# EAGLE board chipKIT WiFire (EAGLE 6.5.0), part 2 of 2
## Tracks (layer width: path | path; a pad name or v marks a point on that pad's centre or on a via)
AETXCLK/RPA14/SCL1/RA14  (via drill 0.23 pad 0.43)
  Top 0.127: v63.63,43.56 63.75,43.43 64.64,43.43 65.02,43.05 65.02,42.04 68.2,38.86 68.2,31.5 66.22,29.52 IC1.66 59.76,29.52 v59.69,29.59 | JP7.2 68.58,15.62 62.23,21.97 v62.23,22.35
  Bottom 0.127: v63.63,43.56 63.75,43.69 63.75,49.02 J7.1 | v59.69,29.59 59.69,29.46 60.2,28.96 60.2,24.38 60.83,23.75 60.83,23.37 61.85,22.35 v62.23,22.35
AETXEN/RPA15/SDA1/RA15  (via drill 0.23 pad 0.43)
  Top 0.127: IC3.33 26.16,32.26 v26.29,32.38 | v57.66,26.92 57.66,29.59 58.17,30.1 59.82,30.1 59.99,29.92 IC1.67
  Bottom 0.127: R21.1 26.42,32.51 v26.29,32.38 27.3,31.37 33.02,31.37 34.04,30.35 38.48,30.35 42.55,26.29 48.51,26.29 48.9,25.91 55.24,25.91 56.39,27.05 57.53,27.05 v57.66,26.92
AN2/C2INB/RPB2/RB2
  Top 0.203: IC1.23 46.42,24.32 45.21,23.11 45.21,19.68 51.82,13.08 54.61,13.08 55.5,12.19 66.04,12.19 71.37,6.86 71.88,6.86 J8.4
AN3/C2INA/RPB3/RB3
  Top 0.203: IC1.22 46.18,24.72 44.7,23.24 44.7,19.56 51.69,12.57 54.23,12.57 55.12,11.68 65.91,11.68 71.12,6.48 J8.2
AN4/C1INB/RB4
  Top 0.203: IC1.21 45.95,25.12 44.2,23.37 44.2,19.3 51.56,11.94 53.72,11.94 54.48,11.18 65.79,11.18 69.22,7.75 69.22,4.32 69.6,3.94 75.06,3.94 J8.6
AN6/ERXERR/AETXERR/RB11  (via drill 0.23 pad 0.43)
  Top 0.127: v82.04,44.32 81.28,43.56 76.96,43.56 v72.77,39.37 | IC1.35 52.9,22.93 53.59,23.62 53.59,27.18 52.9,27.87 52.9,29.28 53.85,30.23 v53.85,30.48
  Bottom 0.127: R25.1 82.05,44.33 v82.04,44.32 | v72.77,39.37 70.48,37.08 61.47,37.08 58.8,34.42 55.24,34.42 54.99,34.16 54.99,31.62 v53.85,30.48
AN8/ERXD1/AECOL/RB13  (via drill 0.23 pad 0.43)
  Top 0.203: v72.14,33.02 71.5,32.38 71.5,26.04 71.12,25.65 71.12,21.21 70.23,20.32 v67.69,20.32 | IC1.42 55.7,22.68 v55.75,22.73
  Bottom 0.203: v72.14,33.02 72.38,33.02 R11.1 | v55.75,22.73 56.26,23.24 60.45,23.24 61.85,21.84 62.99,21.84 64.52,20.32 v67.69,20.32
AN14/C1IND/ECOL/RPG6/SCK2/RG6  (via drill 0.23 pad 0.43)
  Top 0.127: v50.04,30.48 49.08,29.52 IC1.10
  Bottom 0.127: 77.98,44.97 R26.1 78.87,45.85 82.17,45.85 82.93,46.61 84.33,46.61 85.85,48.13 85.85,51.18 84.45,52.58 50.55,52.58 49.28,51.31 J7.11 50.42,49.66 50.42,47.75 49.28,46.61 46.74,46.61 44.83,44.7 44.83,40.51 44.96,40.39 44.96,34.8 48.39,31.37 49.15,31.37 v50.04,30.48 50.55,29.97 52.2,29.97 53.21,28.96 56.77,28.96 57.53,28.19 59.05,28.19 59.31,28.45 59.31,28.83 58.8,29.34 58.8,29.97 59.44,30.61 65.28,30.61 65.91,31.24 76.33,31.24 76.83,31.75 79.38,31.75 83.19,27.94 J9.3
AN23/AERXERR/RG15  (via drill 0.23 pad 0.43)
  Top 0.127: v85.09,45.85 85.34,45.59 85.34,39.12 84.58,38.35 73.03,38.35 71.5,39.88 71.5,41.53 68.83,44.2 58.04,44.2 57.28,43.43 56.39,43.43 v56.01,43.05 | IC1.1 48.29,33.12 v48.51,32.89
  Bottom 0.127: v85.09,45.85 R23.1 | v48.51,32.89 51.44,32.89 52.32,33.78 52.32,35.18 55.24,38.1 55.75,38.1 56.01,38.35 56.01,38.86 55.24,39.62 54.23,39.62 53.34,40.51 53.34,42.16 54.23,43.05 v56.01,43.05
AN25/AERXD0/RPE8/RE8  (via drill 0.23 pad 0.43)
  Top 0.127: v62.23,37.72 62.23,36.45 55.75,29.97 v55.75,28.32 | v50.8,27.56 50.55,27.56 49.31,26.32 IC1.18
  Bottom 0.127: J10.5 77.6,49.66 77.6,47.5 74.93,44.83 74.93,43.94 68.71,37.72 v62.23,37.72 | v55.75,28.32 55.75,28.19 54.61,27.05 51.69,27.05 51.44,27.3 51.05,27.3 v50.8,27.56
AN26/AERXD1/RPE9/RE9  (via drill 0.23 pad 0.43)
  Top 0.127: v64.39,42.93 64.39,42.42 62.74,40.77 62.74,36.45 56.39,30.1 56.39,28.19 v56.26,28.07 | v51.44,26.67 51.31,26.67 50.56,25.92 IC1.19
  Bottom 0.127: v64.39,42.93 64.39,49.15 J10.15 | v56.26,28.07 56.26,27.94 54.99,26.67 v51.44,26.67
AN32/AETXD0/RPD14/RD14  (via drill 0.23 pad 0.43)
  Top 0.127: v54.1,28.07 54.23,27.94 54.23,25.53 56.9,22.86 57.4,22.86 57.7,22.56 IC1.47
  Bottom 0.127: 49.4,48.26 J7.12 49.02,48.26 47.75,46.99 46.35,46.99 44.45,45.09 44.45,40.39 44.58,40.26 44.58,34.67 48.26,30.99 48.9,30.99 50.16,29.72 51.94,29.72 53.09,28.57 53.59,28.57 v54.1,28.07
AN33/AETXD1/RPD15/SCK6/RD15  (via drill 0.23 pad 0.43)
  Top 0.127: v53.47,28.07 53.98,28.57 54.36,28.57 54.61,28.32 54.61,25.78 57.28,23.11 57.53,23.11 58.1,22.54 IC1.48
  Bottom 0.127: J7.14 44.07,45.59 44.07,40.26 44.2,40.13 44.2,34.42 48.01,30.61 48.77,30.61 49.91,29.46 51.69,29.46 53.09,28.07 v53.47,28.07
AN45/C1INA/RPB5/RB5
  Top 0.203: IC1.20 45.59,25.52 43.69,23.62 43.69,19.05 51.44,11.3 52.83,11.3 53.59,10.54 53.59,9.4 54.61,8.38 64.14,8.38 69.98,2.54 J8.1
AVCC
  Top 0.254: IC1.30 50.9,20.8 C15.1
  pour Top (no thermals): 50.29,20.32 50.29,18.67 47.88,18.67 47.88,19.81 49.02,19.81 49.53,20.32
EBIA0/AN10/ERXD3/AETXD2/RPB15/OCFB/PMA0/RB15  (via drill 0.23 pad 0.43)
  Top 0.203: IC1.44 56.5,15.25 57.02,14.73 67.44,14.73 v75.18,6.99
  Bottom 0.203: J8.7 77.47,3.81 77.47,5.84 76.33,6.99 v75.18,6.99
EBIA1/AN9/ERXD2/AETXD3/RPB14/SCK3/PMA1/RB14  (via drill 0.23 pad 0.43)
  Top 0.127: J13.5 20.57,3.3 20.95,2.92 25.15,2.92 26.17,3.94 26.17,15.75 27.94,17.53 32,17.53 32.89,18.41 40.39,18.41 40.64,18.67 41.02,18.67 41.15,18.54 v41.27,18.54 | IC1.43 56.1,20.29 56.01,20.19 56.01,17.65 55.12,16.76 v52.7,16.76
  Bottom 0.127: v41.27,18.54 46.74,18.54 48.51,16.76 v52.7,16.76
EBIA2/AN11/C2INC/ERXCLK/EREFCLK/AERXCLK/AEREFCLK/RPG9/PMA2/RG9  (via drill 0.23 pad 0.43)
  Top 0.127: v50.67,30.48 50.67,29.34 50.29,28.96 50.29,28.07 49.15,26.92 v48.51,26.92 | 48.33,27.11 v48.51,26.92 | IC1.16 48.32,27.12 v48.51,26.92
  Bottom 0.127: J7.5 56.9,51.56 56.39,52.07 51.05,52.07 50.67,51.69 50.67,50.16 51.31,49.53 52.32,49.53 52.83,49.02 52.83,46.99 51.69,45.85 47.5,45.85 45.59,43.94 45.59,39.88 46.1,39.37 46.1,37.21 46.74,36.58 46.74,35.94 47.5,35.18 47.5,32.77 48.39,31.88 49.4,31.88 50.67,30.61 v50.67,30.48 | v48.51,26.92 49.15,26.29 51.05,26.29 51.18,26.16 51.94,26.16 52.07,26.29 55.12,26.29 56.26,27.43 58.8,27.43 59.69,28.32 59.69,28.96 59.18,29.46 59.18,29.84 59.44,30.1 77.09,30.1 77.34,29.84 78.23,29.84 JP5.1 JP5.2 80.9,27.18 82.68,25.4 J9.5
EBIA3/AN12/C2IND/ERXDV/ECRSDV/AERXDV/AECRSDV/RPG8/SCL4/PMA3/RG8  (via drill 0.23 pad 0.43)
  Top 0.127: IC1.12 48.24,28.72 48.39,28.57 48.9,28.57 v49.02,28.45
  Top 0.203: IC1.12 46.34,28.72 46.1,28.96 44.07,28.96 42.55,27.43 42.55,18.29 50.16,10.67 50.16,8.89 51.31,7.75 63.88,7.75 70.36,1.27 79.38,1.27 80.01,1.91 80.01,3.17 80.64,3.81 82.55,3.81 J8.11
  Bottom 0.127: J6.2 39.12,47.12 40.01,46.23 40.01,38.23 42.16,36.07 42.16,29.84 43.18,28.83 45.34,28.83 46.1,28.07 48.64,28.07 v49.02,28.45
EBIA4/AN13/C1INC/ECRS/RPG7/SDA4/PMA4/RG7  (via drill 0.23 pad 0.43)
  Top 0.127: v48.51,29.08 47.44,29.08 IC1.11
  Top 0.203: J8.9 81.28,2.29 79.76,0.76 70.1,0.76 63.75,7.11 51.05,7.11 49.4,8.76 49.4,10.41 41.78,18.03 41.78,27.69 43.43,29.34 46.23,29.34 46.44,29.12 IC1.11
  Bottom 0.127: J6.1 41.66,47.24 40.39,45.97 40.39,38.35 42.55,36.2 42.55,30.35 43.81,29.08 45.72,29.08 46.35,28.45 48.26,28.45 48.51,28.7 v48.51,29.08
EBIA5/AN34/PMA5/RA5  (via drill 0.23 pad 0.43)
  Top 0.127: IC1.2 43.77,32.72 40.51,29.46 40.51,24.77 v39.88,24.13
  Bottom 0.127: R27.1 25.03,25.53 31.62,25.53 32,25.91 33.78,25.91 34.04,25.65 38.35,25.65 v39.88,24.13
EBIA6/AN22/RPC1/PMA6/RC1  (via drill 0.23 pad 0.43)
  Top 0.127: IC1.6 48.52,31.12 48.77,31.37 53.98,31.37 54.74,32.13 57.28,32.13 57.91,32.77 58.17,32.77 60.45,35.05 60.45,35.69 61.59,36.83 61.59,42.93 61.72,43.05 v61.72,43.31
  Bottom 0.127: J7.4 59.44,48.64 60.33,49.53 62.23,49.53 63.12,48.64 63.12,45.21 61.72,43.81 v61.72,43.31
EBIA7/AN49/RPB9/PMA7/RB9  (via drill 0.23 pad 0.43)
  Top 0.203: IC1.33 52.1,16.61 53.59,15.11 55.75,15.11 56.64,14.22 67.06,14.22 v69.09,12.19
  Bottom 0.203: v69.09,12.19 74.93,6.35 74.93,3.81 J8.3
EBIA8/RPF5/SCL5/PMA8/RF5  (via drill 0.23 pad 0.43)
  Top 0.127: IC3.32 24.89,30.86 26.29,29.46 v27.81,29.46 | v57.91,25.91 57.91,26.04 58.42,26.54 58.42,28.19 58.29,28.32 58.29,28.83 58.59,29.12 IC1.65
  Bottom 0.127: v27.81,29.46 30.61,29.46 32.51,27.56 34.92,27.56 35.18,27.3 36.45,27.3 36.96,27.81 38.86,27.81 41.53,25.15 55.5,25.15 56.39,26.04 57.78,26.04 v57.91,25.91
EBIA9/RPF4/SDA5/PMA9/RF4  (via drill 0.23 pad 0.43)
  Top 0.127: IC3.7 22.35,51.56 v22.1,51.31 22.1,51.05 22.61,50.55 27.18,50.55 29.46,48.26 34.8,48.26 35.94,47.12 43.31,47.12 45.09,45.34 v48.01,45.34 | v58.8,28.7 60.78,28.7 IC1.64
  Bottom 0.127: v22.1,51.31 R14.1 | v48.01,45.34 48.01,39.12 50.67,36.45 50.67,33.66 50.29,33.27 49.02,33.27 48.77,33.53 48.13,33.53 47.88,33.27 47.88,32.89 48.51,32.26 50.42,32.26 53.34,29.34 57.66,29.34 58.29,28.7 v58.8,28.7
EBIA10/AN48/RPB8/PMA10/RB8
  Top 0.203: IC1.32 51.7,16.24 53.34,14.61 55.5,14.61 56.39,13.72 66.8,13.72 74.17,6.35 80.64,6.35 81.28,5.71 J8.10
EBIA11/AN7/ERXD0/AECRS/PMA11/RB12  (via drill 0.23 pad 0.43)
  Top 0.127: IC1.41 55.3,20.77 55.75,20.32 55.75,17.91 54.99,17.14 53.85,17.14 53.59,17.4 v53.09,17.4 | v43.69,15.24 40.13,15.24 39.5,15.88 35.81,15.88 32,12.06 v32,10.67
  Bottom 0.127: v53.09,17.4 53.09,17.27 53.21,17.14 53.21,16 52.45,15.24 v43.69,15.24 | v32,10.67 R35.1
  Bottom 0.203: R36.2 R35.1
EBIA12/AN21/RPC2/PMA12/RC2  (via drill 0.23 pad 0.43)
  Top 0.203: IC1.7 49.26,30.72 49.53,30.99 54.1,30.99 55.12,29.97 55.12,26.04 58.42,22.73 60.07,22.73 65.91,16.89 v65.91,15.37
  Bottom 0.203: v65.91,15.37 67.94,13.34 69.72,13.34 74.93,8.13 76.58,8.13 78.36,6.35 79.5,6.35 80.01,5.84 80.01,1.91 79.38,1.27 77.47,1.27 J8.5
EBIA13/CVREFOUT/AN5/RPB10/PMA13/RB10  (via drill 0.23 pad 0.43)
  Top 0.127: J13.7 18.29,4.89 18.29,3.43 19.3,2.41 25.65,2.41 28.37,5.13 28.37,15.29 30.1,17.02 40.01,17.02 v40.89,17.91 | IC1.34 52.5,18.87 v52.58,18.8
  Bottom 0.127: v40.89,17.91 40.77,18.03 40.77,18.8 41.02,19.05 46.99,19.05 48.01,18.03 51.82,18.03 v52.58,18.8
EBIA14/PMCS1/PMA14/RA4  (via drill 0.23 pad 0.43)
  Top 0.127: v57.66,24.64 58.17,25.15 58.17,25.53 58.42,25.78 58.42,26.04 58.67,26.29 58.67,27.18 59.02,27.52 IC1.61
  Bottom 0.127: v57.66,24.64 56.64,23.62 49.66,23.62 49.53,23.75 48.51,23.75 48.39,23.62 39.75,23.62 38.35,25.02 34.8,25.02 34.66,24.88 R29.1
EBIA15/RPD9/PMCS2/PMA15/RD9  (via drill 0.23 pad 0.43)
  Top 0.127: v13.46,32.38 IC3.23 13.5,31.71 14.22,30.99 19.18,30.99 23.11,27.05 v23.88,27.05 | v56.52,25.53 56.52,25.65 57.28,26.42 57.28,26.67 57.15,26.8 57.15,29.59 57.91,30.35 59.94,30.35 59.98,30.32 IC1.68
  Bottom 0.127: v13.46,32.38 13.46,33.01 R20.1 | v23.88,27.05 38.99,27.05 41.27,24.77 55.63,24.77 56.39,25.53 v56.52,25.53
EBICS0/SCL2/RA2  (via drill 0.23 pad 0.43)
  Top 0.127: v58.29,29.59 58.04,29.34 58.04,27.56 58.17,27.43 58.17,26.8 57.78,26.42 57.66,26.42 57.15,25.91 57.15,24.51 57.53,24.13 57.91,24.13 58.55,24.77 58.55,25.53 58.8,25.78 58.8,26.04 58.93,26.16 58.93,26.54 59.11,26.72 IC1.59
  Bottom 0.127: J7.8 56.52,46.1 56.52,42.8 55.37,41.66 55.37,40.01 56.39,38.99 56.39,38.35 55.88,37.85 55.5,37.85 54.74,37.08 54.74,36.45 52.96,34.67 52.96,33.66 52.07,32.77 52.07,31.11 53.47,29.72 58.17,29.72 v58.29,29.59
EBID0/PMD0/RE0
  Top 0.127: J10.2 81.79,46.23 78.11,46.23 76.45,44.58 56.52,44.58 55.5,43.56 55.5,42.55 55.75,42.29 55.75,40.51 53.09,37.85 53.09,36.32 52.9,36.14 IC1.91
EBID1/PMD1/RE1
  Top 0.127: J10.4 79.63,46.61 77.85,46.61 76.33,45.09 56.39,45.09 55.12,43.81 55.12,42.42 55.37,42.16 55.37,40.64 52.7,37.97 51.82,37.97 51.05,37.21 51.05,36.45 51.31,36.2 51.56,36.2 51.7,36.05 IC1.94
EBID2/PMD2/RE2
  Top 0.127: 76.07,45.59 77.22,46.74 77.47,46.74 78.74,48.01 J10.6 | 50.67,45.59 48.9,43.81 46.35,43.81 45.47,42.93 45.47,40.01 47.62,37.85 48.39,37.85 49.78,36.45 49.78,36.2 50.1,35.88 IC1.98
  Top 0.203: 50.67,45.59 76.07,45.59
EBID3/RPE3/PMD3/RE3
  Top 0.127: J10.8 76.2,47.5 74.8,46.1 50.42,46.1 48.51,44.2 46.1,44.2 44.83,42.93 44.83,40.13 47.62,37.34 48.26,37.34 49.7,35.9 IC1.99
EBID4/AN18/PMD4/RE4
  Top 0.127: J10.10 73.66,47.24 73.03,46.61 50.29,46.61 48.39,44.7 45.85,44.7 44.45,43.31 44.45,40.01 47.62,36.83 48.26,36.83 49.3,35.79 IC1.100
EBID5/AN17/RPE5/PMD5/RE5  (via drill 0.23 pad 0.43)
  Top 0.127: v52.96,32.51 52.77,32.32 IC1.3
  Bottom 0.127: J10.12 70.74,47.88 70.74,43.81 67.44,40.51 63.5,40.51 57.78,34.8 55.12,34.8 54.23,33.91 54.23,32.38 53.85,32 53.47,32 v52.96,32.51
EBID6/AN16/PMD6/RE6  (via drill 0.23 pad 0.43)
  Top 0.127: IC1.4 48.43,31.92 48.51,32 53.21,32 v53.72,32.51
  Bottom 0.127: J10.14 67.82,47.5 67.82,43.31 66.17,41.66 63.12,41.66 60.2,38.73 57.78,38.73 56.9,37.85 56.9,36.32 55.75,35.18 54.86,35.18 53.72,34.04 v53.72,32.51
EBID7/AN15/PMD7/RE7  (via drill 0.23 pad 0.43)
  Top 0.127: v60.07,39.88 59.69,39.5 59.69,34.67 58.04,33.02 57.15,33.02 56.64,32.51 54.61,32.51 53.85,31.75 48.64,31.75 48.41,31.52 IC1.5
  Bottom 0.127: v60.07,39.88 62.61,42.42 64.64,42.42 65.15,42.93 65.15,47.37 J10.16
EBID8/RPG0/PMD8/RG0
  Top 0.127: IC1.88 54.1,34.16 53.98,34.04 53.98,33.91 53.85,33.78 52.2,33.78 51.82,33.4 49.78,33.4 48.9,34.29 48.9,34.54 42.04,41.4 36.83,41.4 35.05,43.18 31.5,43.18 28.57,40.26 28.57,31.84 IC3.35
EBID9/ETXERR/RPG1/PMD9/RG1  (via drill 0.23 pad 0.43)
  Top 0.127: IC3.20 v9.65,32.38 11.43,34.16 27.69,34.16 28.07,33.78 28.07,31.11 28.32,30.86 30.35,30.86 30.86,31.37 30.86,39.24 32.51,40.89 38.35,40.89 41.78,37.47 43.94,37.47 44.07,37.59 44.83,37.59 47.5,34.92 47.88,34.92 49.66,33.15 51.94,33.15 52.32,33.53 54.1,33.53 54.5,33.93 IC1.87
  Bottom 0.127: R19.1 v9.65,32.38
EBID10/ETXD0/RPF1/PMD10/RF1  (via drill 0.23 pad 0.43)
  Top 0.127: IC1.86 54.9,35.78 54.61,36.07 54.36,36.07 53.98,36.45 53.98,37.72 56.01,39.75 57.28,39.75 58.04,40.51 58.04,41.78 v57.66,42.16
  Bottom 0.127: J7.6 56.9,47.62 57.66,46.86 57.66,43.18 57.4,42.93 57.4,42.42 v57.66,42.16
EBID11/ETXD1/RPF0/PMD11/RF0  (via drill 0.23 pad 0.43)
  Top 0.127: v55.5,38.61 54.48,37.59 54.48,36.7 55.3,35.88 IC1.85 55.3,34.11 v55.5,33.91
  Bottom 0.127: J7.9 51.94,50.8 53.21,49.53 53.21,43.81 52.96,43.56 52.96,40.26 53.98,39.24 54.86,39.24 v55.5,38.61 | J9.1 81.41,30.48 79.63,32.26 76.07,32.26 75.44,31.62 64.52,31.62 63.88,30.99 61.34,30.99 60.33,32 56.52,32 55.5,33.02 v55.5,33.91
EBID12/ETXD2/RPD12/PMD12/RD12  (via drill 0.23 pad 0.43)
  Top 0.127: v46.99,33.78 48.26,33.78 49.4,32.64 52.2,32.64 52.58,33.02 56.64,33.02 57.02,33.4 57.4,33.4 57.7,33.7 IC1.79
  Bottom 0.127: J7.10 49.78,46.23 46.99,46.23 45.21,44.45 45.21,40.64 45.34,40.51 45.34,37.47 45.72,37.08 45.72,34.67 46.61,33.78 v46.99,33.78
EBID13/ETXD3/PMD13/RD13  (via drill 0.23 pad 0.43)
  Top 0.127: IC1.80 57.3,34.06 56.77,33.53 55.75,33.53 55.63,33.4 54.36,33.4 54.23,33.27 52.45,33.27 52.07,32.89 49.53,32.89 48.13,34.29 43.69,34.29 39.37,29.97 39.37,21.34 v40.26,20.45
  Bottom 0.127: R37.1 50.29,7.37 50.29,9.65 48.64,11.3 46.86,11.3 40.26,17.91 v40.26,20.45
EBID14/ETXEN/RPD2/PMD14/RD2  (via drill 0.23 pad 0.43)
  Top 0.127: v58.93,39.24 58.67,38.99 58.67,36.07 58.5,35.9 IC1.77
  Bottom 0.127: v58.93,39.24 59.05,39.12 60.07,39.12 62.99,42.04 65.41,42.04 66.55,43.18 66.55,46.74 67.31,47.5 67.31,49.53 J10.13
EBID15/ETXCLK/RPD3/PMD15/RD3  (via drill 0.23 pad 0.43)
  Top 0.127: IC1.78 58.1,35.88 58.29,36.07 58.29,40.13 58.42,40.26 58.42,42.29 v58.17,42.55
  Bottom 0.127: J7.3 59.31,50.8 58.17,49.66 v58.17,42.55
EBIOE/AN19/RPC4/PMRD/RC4
  Top 0.127: J13.3 22.77,4.03 23.24,3.56 25.27,3.56 25.78,4.06 25.78,16.26 27.69,18.16 31.75,18.16 32.51,18.92 40.13,18.92 41.27,20.07 41.27,28.45 42.75,29.92 IC1.9
EBIRDY1/SDA2/RA3  (via drill 0.23 pad 0.43)
  Top 0.127: IC1.60 61.78,27.12 61.98,26.92 66.29,26.92 69.22,29.84 69.22,34.29 68.96,34.54 v68.96,40.51
  Bottom 0.127: J10.9 72.39,49.53 72.39,44.7 68.96,41.27 v68.96,40.51
EBIRDY2/RPF8/SCL3/RF8  (via drill 0.23 pad 0.43)
  Top 0.127: v59.69,26.29 60.77,26.29 IC1.58 61.63,26.32 61.85,26.54 66.55,26.54 69.85,29.84 69.85,33.53 70.99,34.67 75.56,34.67 76.2,35.31 76.2,37.47 v75.82,37.85
  Bottom 0.127: R8.2 20.45,18.29 21.46,19.3 21.46,21.46 21.72,21.72 21.72,25.15 22.73,26.16 38.48,26.16 40.64,24 56.26,24 57.4,25.15 59.31,25.15 59.82,25.65 59.82,26.16 v59.69,26.29 | J10.3 80.01,49.53 80.01,47.62 79.25,46.86 77.72,46.86 75.69,44.83 75.69,37.97 v75.82,37.85
EBIRDY3/RPF2/SDA3/RF2  (via drill 0.23 pad 0.43)
  Top 0.127: v59.31,25.78 59.82,25.78 59.94,25.91 60.79,25.91 IC1.57 61.73,25.92 61.98,26.16 66.8,26.16 70.36,29.72 70.36,32.38 71.75,33.78 75.69,33.78 76.71,34.8 v76.71,37.85
  Bottom 0.127: J10.1 82.55,49.53 82.55,47.62 81.28,46.35 77.98,46.35 76.2,44.58 76.2,41.02 76.71,40.51 v76.71,37.85 | R7.2 18.04,20.58 19.18,21.72 20.7,21.72 21.08,22.1 21.08,25.27 22.35,26.54 38.86,26.54 41.02,24.38 56.13,24.38 57.15,25.4 58.93,25.4 v59.31,25.78
EBIWE/AN20/RPC3/PMWR/RC3
  Top 0.127: J13.2 24.13,5.63 24.13,5.97 25.02,6.86 25.02,16.26 24.51,16.76 22.61,16.76 22.48,16.89 R22.1 22.6,17.53 25.91,17.53 27.3,18.92 31.75,18.92 32.26,19.43 40.01,19.43 40.89,20.32 40.89,28.7 42.51,30.32 IC1.8
EMDC/AEMDC/RPD11/RD11  (via drill 0.23 pad 0.43)
  Top 0.127: v66.55,30.73 66.17,30.35 63.63,30.35 63.25,30.73 62.74,30.73 62.35,31.12 IC1.70 v59.69,31.11
  Bottom 0.127: v66.55,30.73 76.71,30.73 77.09,31.11 79.12,31.11 81.66,28.57 81.66,27.94 82.8,26.8 85.22,26.8 J9.4 | J7.7 54.48,50.8 55.63,49.66 55.63,47.88 56.9,46.61 56.9,42.67 55.88,41.66 55.88,40.01 56.77,39.12 56.77,38.35 56.01,37.59 55.63,37.59 55.12,37.08 55.12,36.07 53.34,34.29 53.34,33.53 52.45,32.64 52.45,31.62 53.34,30.73 53.34,30.35 53.72,29.97 54.23,29.97 55.37,31.11 v59.69,31.11
EMDIO/AEMDIO/RPD0/RTCC/INT0/RD0  (via drill 0.23 pad 0.43)
  Top 0.127: v67.56,38.35 67.06,37.85 67.06,33.15 65.02,31.11 62.87,31.11 62.46,31.52 IC1.71
  Bottom 0.127: J10.7 75.06,49.66 75.06,47.24 73.91,46.1 73.91,44.7 v67.56,38.35
FT3V3  (via drill 0.23 pad 0.43)
  Top 0.508: 12.32,25.02 12.32,22.61 12.95,21.97 14.86,21.97 v16.26,20.57 | 12.32,25.02 12.57,25.27 12.57,26.8 11.94,27.43 11.94,29.59 12.83,30.48 v15.75,30.48 v16.76,30.48 | 12.32,25.02 11.05,25.02 v10.16,25.91
  Bottom 0.127: R9.2 v16.76,30.48 | R10.2 v15.75,30.48
  Bottom 0.254: IC2.16 10.96,25.63 C13.1 v10.17,25.92 v10.16,25.91 | IC2.1 15.72,20.59 C11.1 16.25,20.57 v16.26,20.57
GND  (via drill 0.23 pad 0.43)
  Top 0.127: C20.2 v63,31.76 v62.99,31.75 | C19.2 v63,34.79 v62.99,34.8
  Top 0.203: IC7.2 61.66,16.58 61.72,16.51
  Top 0.254: IC3.30 22.35,31.5 22.1,31.24 C21.2 21.84,30.23 v21.84,29.97 | IC3.18 8.38,51.94 8.64,51.69 v8.64,51.56 | IC3.10 v18.54,51.44 | IC3.1 v29.97,51.44 | IC3.19 v8.38,32.38 | IC3.25 v16,32.38 | IC3.28 v19.81,32.38 | IC3.36 v29.97,32.38 | C15.2 | C15.2 v51.05,19.44 v51.05,19.43 | C14.2 51.05,18.79 v50.8,18.54 | C15.2 51.05,20.31 51.3,20.57 IC1.31 | C6.2 | C6.2 v53.09,19.44 v53.09,19.43 | C8.2 | v19.94,3.68 19.47,4.15 J13.6 | v52.32,37.08 52.32,36.95 C3.2 52.5,36.63 IC1.92 | IC1.84 55.7,36.51 C2.2 55.75,36.95 v55.75,37.08 | IC1.53 62.41,24.32 C1.2 62.73,24 v62.99,24 | IC1.63 62.24,28.32 C10.2 62.73,28.32 v62.99,28.32 | IC1.13 45.84,28.32 C4.2 45.6,28.32 v45.21,28.32 | IC1.36 53.3,20.15 C6.2 | IC1.45 56.9,20.07 C8.2 | 61.59,33.15 v61.72,33.27 61.57,33.12 IC1.75 | C8.2 v57.02,19.43
  Top 0.305: v62.23,16.51 61.72,16.51 | C17.2 v57.78,16.38
  Top 1.27: 5.08,20.19 J1.S3 J1.S2 5.08,29.09 | 5.08,20.19 J1.S4 | J1.S1 5.08,29.09 | J1.S5 5.08,29.09 | J1.S6 5.08,20.19
  Route2 1.524: 4.32,12.19 J15.2 4.32,4.45 5.84,2.92 J15.3
  Bottom 0.127: C5.2 R2.1 v10.67,29.46 | R30.1 v23.37,25.4 | R32.1 v32.77,25.4 | R15.1 v13.2,51.3 v13.21,51.31 | R17.1 v79.49,15.76 v79.5,15.75
  Bottom 0.203: Q2.1 v79.12,42.55 | Q2.4 80.45,44.13 v80.52,44.2
  Bottom 0.254: IC2.24 15.72,26.52 v15.88,26.67 | IC2.26 16.74,25.13 v16.76,25.15 | C13.2 v10.17,26.92 v10.16,26.92 | IC2.4 v14.22,21.09 v14.22,21.08 | C11.2 16,19.81 v16.13,19.81 | IC2.17 11.97,26.13 v11.81,26.29 | R41.1 v35.31,22.1 | IC2.20 13.72,26.94 C9.2 13.96,27.68 v13.97,27.69 | C7.2 14.35,28.7 | 14.35,28.7 v13.97,28.32 | C23.2 v8.64,51.55 v8.64,51.56 | D2.2 v31.5,41.02 | R36.1 31.11,8.89 v31.88,8.13 | 14.35,28.7 14.35,28.83 14.1,29.08 v13.97,29.08 | Q1.1 v83.19,42.55 | Q1.4 84.52,44.13 v84.58,44.2 | v19.68,48.77 19.68,49.13 C25.2 18.92,49.16 v18.92,48.77 | v4.7,33.53 4.7,33.92 C26.2 5.08,34.29 5.46,33.91 v5.46,33.53 | C27.2 20.07,3.55 v19.94,3.68 | D1.1 50.78,28.21 v50.8,28.19 | C12.2 61.46,33.27 v61.72,33.27
  Bottom 1.27: J11.S3 J11.S1 J11.S2 J11.S4 87.25,13.27 v87.25,11.18
  other vias: 6.48,22.48 6.99,21.97 85.22,15.24 84.2,15.24 13.21,24.64 14.73,24.64 13.21,23.11 14.73,23.11 7.49,22.48 8,21.97 8.51,22.48 13.34,10.92 13.34,11.94 13.34,12.95 13.34,13.72 13.34,14.61 14.22,10.92 14.22,11.94 14.22,12.95 22.73,7.24 22.73,6.48 23.75,6.48 32.26,20.45 32.77,20.07 33.4,20.45 33.15,17.78 34.04,17.78 36.83,17.91 36.07,17.91 37.85,14.99 37.85,13.97 35.31,17.91 37.34,14.48 37.34,13.34 37.85,12.95 37.34,12.32 67.94,25.65 67.94,26.29 83.57,15.75 83.57,14.61 84.84,14.61 81.03,14.22 81.03,13.34 80.52,18.54 81.92,18.54 86.87,11.81 87.63,11.81
  pour Top (no thermals): 6.22,23.37 9.02,23.37 9.02,21.72 6.22,21.72
  pour Bottom (no thermals): 85.47,16 83.06,16 83.06,14.22 85.47,14.22
  pour Top (no thermals): 5.21,5.59 5.21,9.65 4.7,10.16 3.94,10.16 3.43,9.65 3.43,5.59 3.94,5.08 4.7,5.08
  pour Top (no thermals): 5.33,2.03 9.4,2.03 9.91,2.54 9.91,3.3 9.4,3.81 5.33,3.81 4.83,3.3 4.83,2.54
  pour Bottom (no thermals): 3.43,9.65 3.94,10.16 4.7,10.16 5.21,9.65 5.21,5.59 4.7,5.08 3.94,5.08 3.43,5.59
  pour Bottom (no thermals): 4.83,3.3 5.33,3.81 9.4,3.81 9.91,3.3 9.91,2.54 9.4,2.03 5.33,2.03 4.83,2.54
  pour Bottom (isolate 0.305, rank 2, no thermals): 13.08,9.27 15.11,9.27 15.11,14.99 13.08,14.99
  pour Bottom (no thermals): 22.48,7.49 22.61,7.62 24,7.62 24,5.59 22.48,5.59
  pour Bottom (isolate 0.305, rank 2, no thermals): 32,22.48 32,19.81 32.77,19.81 32.89,19.68 32.89,17.14 37.21,17.14 37.34,17.02 37.34,14.73 37.21,14.61 35.05,14.61 35.05,12.19 38.61,12.19 38.61,18.29 37.08,19.81 35.18,19.81 35.18,18.41 34.92,18.16 33.78,18.16 33.66,18.29 33.66,22.48
  pour Route2 (isolate 0.305): 12.57,0 12.57,11.18 0,11.18 0,35.94 11.81,35.94 11.81,50.93 8.26,50.93 8.26,53.34 88.9,53.34 88.9,0
  pour Route2 (no thermals): 3.43,9.65 3.94,10.16 4.7,10.16 5.21,9.65 5.21,5.59 4.7,5.08 3.94,5.08 3.43,5.59
  pour Route2 (no thermals): 4.83,2.54 4.83,3.3 5.33,3.81 9.4,3.81 9.91,3.3 9.91,2.54 9.4,2.03 5.33,2.03
  pour Bottom (rank 2, no thermals): 68.2,25.4 68.2,26.42 66.93,26.42 66.93,25.4
  pour Bottom (no thermals): 80.64,14.73 80.64,12.7 82.55,12.7 82.55,14.73
  pour Bottom (rank 2, no thermals): 80.14,18.92 80.14,18.16 82.17,18.16 82.17,18.92
  pour Route15 (no thermals): 5.21,5.59 5.21,9.65 4.7,10.16 3.94,10.16 3.43,9.65 3.43,5.59 3.94,5.08 4.7,5.08
  pour Route15 (no thermals): 5.33,2.03 9.4,2.03 9.91,2.54 9.91,3.3 9.4,3.81 5.33,3.81 4.83,3.3 4.83,2.54
N$1
  Bottom 0.406: C24.1 JP6.1
N$14
  Bottom 0.127: C16.2 17.78,23.87 17.78,29.46 22.23,33.91 24.89,33.91 26.16,35.18 29.97,35.18 30.35,35.56 35.69,35.56 36.96,34.29 39.37,34.29 JP2.2
N$17
  Top 0.203: IC1.49 58.5,20.62 59.05,20.07 60.83,20.07 61.38,19.52 IC7.3
N$18
  Top 0.127: X2.2 65.79,33.91 65.41,34.29 64.9,34.29 64.64,34.04 64.64,33.4 64.26,33.02 63.76,33.02 C20.1 62.99,32.26 62.87,32.26 62.48,31.88 61.47,31.88 61.42,31.92 IC1.72
N$19
  Top 0.127: IC1.73 61.53,32.32 61.72,32.13 62.36,32.13 62.48,32.26 R13.2
N$20
  Top 0.127: X2.1 65.79,35.05 65.41,34.67 64.77,34.67 64.26,34.16 64.26,33.53 64.14,33.4 63.88,33.4 C19.1 62.5,33.79 R13.1
N$21  (via drill 0.23 pad 0.43)
  Top 0.127: IC1.15 46.44,27.52 v46.35,27.43
  Bottom 0.127: D1.3 46.48,27.56 v46.35,27.43 46.1,27.18 44.96,27.18 44.32,27.81 R4.1
N$22
  Bottom 0.127: R24.2 79.63,44.58 79.63,43.43 79.88,43.18 Q2.5
N$23
  Bottom 0.127: Q2.3 77.85,43.81 77.6,43.56 77.6,40.64 78.49,39.75 79.5,39.75 79.76,40.01 79.76,40.64 R33.1
N$25
  Bottom 0.127: R16.1 82.04,16.26 82.04,16.89 81.34,17.59 IC4.3 80.33,17.59 79.63,18.29 77.6,18.29 76.58,19.3 69.98,19.3 JP7.1
N$26  (via drill 0.23 pad 0.43)
  Top 0.127: v80.9,40.77 80.9,41.01 LD2.C
  Bottom 0.127: R33.2 v80.9,40.77
N$27
  Bottom 0.127: BTN3.1B 38.14,39.54 38.23,39.62 R6.1 37.47,40.64 37.08,41.02 37.08,44.11 BTN3.2B
N$28  (via drill 0.23 pad 0.43)
  Top 0.127: LD1.C 78.75,41.39 79.12,41.02 v79.12,40.77
  Bottom 0.127: v79.12,40.77 v79.11,40.77 R34.2
N$29  (via drill 0.23 pad 0.43)
  Top 0.127: IC3.26 17.27,31.75 16.89,32.13 v16.89,32.51
  Bottom 0.127: v16.89,32.51 16.89,32.65 R18.1
N$30
  Bottom 0.127: J17.5 49.28,7.37 R37.2
N$31
  Bottom 0.127: Q2.2 79.12,43.18 79.25,43.31 79.25,44.7 R26.2
N$32
  Bottom 0.127: 80.26,42.55 Q2.6 80.39,42.55 79.24,41.39 R34.1
N$33  (via drill 0.23 pad 0.43)
  Top 0.254: J1.2 9.11,25.44 v9.14,25.4
  Bottom 0.254: IC2.15 9.93,25.13 9.65,25.4 v9.14,25.4
N$34
  pour Bottom (rank 2, no thermals): 23.62,17.65 23.62,14.61 28.7,14.61 30.99,12.32 33.02,12.32 33.02,14.61 32.64,14.61 32.64,16.64 31.5,16.64 31.24,16.38 30.23,16.38 29.97,16.64 29.97,17.4 29.72,17.65
N$35
  Bottom 0.305: 30.75,16.89 C30.1 D5.C | 32.32,18.73 31.88,18.29 30.75,18.29
  Bottom 0.508: IC5.1 32.32,18.73 | 30.75,18.29 D5.C
N$36
  pour Bottom (isolate 0.305, rank 2, no thermals): 20.57,6.86 22.1,6.86 22.1,7.62 22.48,8 24,8 24,10.29 22.86,10.29 22.86,9.53 22.61,9.27 20.57,9.27
N$37  (via drill 0.23 pad 0.43)
  Top 0.254: J1.3 9.14,24.64 v9.27,24.77
  Bottom 0.254: IC2.14 9.41,24.63 v9.27,24.77
N$38
  Bottom 0.254: IC5.3 34.22,19.62 34.29,19.68 R40.1 R41.2
N$39
  pour Bottom (isolate 0.305, rank 3, no thermals): 17.78,3.56 17.78,8.64 17.4,9.02 13.08,9.02 13.08,3.56
N$40
  Bottom 0.203: R11.2 VR1.2
N$41
  Bottom 0.127: IC2.30 18.02,23.13 18.29,22.86 18.29,22.34 R7.1
N$43
  Bottom 0.127: IC2.2 15.22,21.06 15.11,20.95 15.11,19.18 15.49,18.8 R8.1
N$45  (via drill 0.23 pad 0.43)
  Top 0.127: IC3.16 10.92,52.07 v11.81,51.18
  Bottom 0.127: v11.81,51.18 v11.82,51.18 R15.2
N$47
  Bottom 0.127: IC2.18 12.72,26.4 12.19,26.92 12.19,27.44 C5.1 R2.2 9.67,28.95 R1.1
N$51  (via drill 0.23 pad 0.43)
  Top 0.127: LD3.C 82.68,41.02 v82.68,40.77
  Bottom 0.127: v82.68,40.77 82.67,40.77 R31.2
N$52
  Bottom 0.127: IC2.8 12.22,20.73 10.54,19.05 7.87,19.05 J4.1
N$53
  Bottom 0.127: IC2.31 17.51,22.63 C16.1
N$54
  Bottom 0.127: IC2.6 13.22,18.43 12.7,17.91 12.7,16.76 12.06,16.13 9.78,16.13 J4.2
N$55
  Bottom 0.127: IC2.7 12.72,18.56 11.43,17.27 J4.3
N$56
  Bottom 0.127: IC2.3 14.72,17.77 14.22,17.27 J4.4
N$57  (via drill 0.23 pad 0.43)
  Top 0.127: v15.75,27.56 15.86,27.56 LD5.C
  Bottom 0.127: IC2.22 14.72,26.53 v15.75,27.56
N$58  (via drill 0.23 pad 0.43)
  Top 0.127: v14.99,27.56 LD6.C
  Bottom 0.127: IC2.21 14.22,26.54 14.99,27.3 v14.99,27.56
N$59  (via drill 0.23 pad 0.43)
  Top 0.127: v17.14,29.34 16.88,29.34 LD5.A
  Bottom 0.127: R9.1 16.77,28.96 v17.14,29.34
N$60  (via drill 0.23 pad 0.43)
  Top 0.127: v15.37,29.21 15.37,29.32 LD6.A
  Bottom 0.127: R10.1 15.61,28.96 v15.37,29.21
N$62
  Bottom 0.127: IC4.4 78.49,17.28 R17.2 77.85,16.26 77.6,16 77.6,15.49 76.96,14.86 74.68,14.86 JP8.1
N$63  (via drill 0.23 pad 0.43)
  Top 0.127: LD4.C 84.09,41.39 84.45,41.02 v84.45,40.77
  Bottom 0.127: v84.45,40.77 R28.2
N$64
  Bottom 0.127: Q1.6 84.33,42.55 83.82,42.04 82.94,42.04 R31.1
N$65
  Bottom 0.127: Q1.3 82.17,43.81 81.92,43.56 81.92,42.42 81.53,42.04 81.53,40.13 81.92,39.75 82.93,39.75 83.19,40.01 83.19,40.51 R28.1
N$66
  Bottom 1.016: J12.1 78.47,13.52 C22.1
  pour Route15 (isolate 0.305, no thermals): 71.75,23.11 71.12,22.48 71.12,20.95 73.03,19.05 73.03,14.73 75.18,12.57 76.96,12.57 76.96,14.48 75.95,14.48 75.31,15.11 75.31,19.68 73.79,21.21 73.79,22.48 73.15,23.11
N$67
  Bottom 0.127: Q1.2 83.06,43.18 83.31,43.43 83.31,44.7 R25.2
N$69
  Bottom 0.127: R23.2 83.69,44.58 83.69,43.43 83.95,43.18 Q1.5
N$71
  Bottom 0.127: 32.74,23.91 R32.2 | R32.2 R29.2 33.81,23.91 BTN2.2A | BTN2.1A 29.29,23.88 R32.2
N$72  (via drill 0.23 pad 0.43)
  Top 0.127: v22.73,23.88 19.9,23.88 BTN1.1A
  Bottom 0.127: v22.73,23.88 22.77,23.91 23.34,23.91 R30.2 R27.2 24.41,23.91 BTN1.2A
P32_PGC  (via drill 0.23 pad 0.43)
  Top 0.127: v37.85,24 37.85,30.48 35.56,32.77 35.56,35.1 JP1.5 | IC1.26 49.3,20.73 v49.28,20.7
  Bottom 0.127: D2.5 30.85,39.64 33.27,37.21 33.45,37.21 JP1.5 | v37.85,24 37.85,23.75 39.24,22.35 48.26,22.35 48.64,21.97 48.95,21.97 IC1.26 49.3,20.73 v49.28,20.7
P32_PGD  (via drill 0.23 pad 0.43)
  Top 0.127: JP1.4 34.42,39.37 36.2,37.59 36.2,33.02 38.35,30.86 v38.35,24.38 | v48.77,22.61 48.9,22.73 49.53,22.73 49.7,22.56 IC1.27
  Bottom 0.127: D2.4 33.87,39.74 JP1.4 | v38.35,24.38 38.35,23.88 39.24,22.99 48.39,22.99 v48.77,22.61
P32_RST  (via drill 0.23 pad 0.43)
  Top 0.127: JP2.1 38.1,33.78 38.99,32.89 v38.99,20.32
  Bottom 0.127: JP1.1 32.38,45.54 32.38,41.91 32.15,41.67 D2.3 32.15,41.51 33.02,40.64 35.94,40.64 36.45,40.13 36.45,36.2 37.08,35.56 JP2.1 | v38.99,20.32 38.99,18.54 46.61,10.92 46.61,9.27 46.86,9.02 46.86,6.6 48.9,4.57 50.8,4.57 52.83,2.54 J5.3 | R4.2 42.8,27.81 41.78,28.83 41.78,35.94 40.89,36.83 40.26,36.83 38.99,35.56 JP2.1 | JP2.1 38.1,36.7 39.23,37.84 R6.2 R5.1
PGEC1/AN1/RPB1/RB1  (via drill 0.23 pad 0.43)
  Top 0.203: IC1.24 46.53,23.92 45.59,22.99 45.59,19.94 51.94,13.59 54.86,13.59 55.75,12.7 v66.29,12.7
  Bottom 0.203: v66.29,12.7 69.47,12.7 74.55,7.62 76.33,7.62 78.74,5.21 J8.8
PGED1/AN0/RPB0/RB0  (via drill 0.23 pad 0.43)
  Top 0.203: IC1.25 46.76,23.52 46.1,22.86 46.1,20.19 52.2,14.1 55.12,14.1 56.01,13.21 66.55,13.21 67.06,12.7 v67.06,12.06
  Bottom 0.203: v67.06,12.06 67.06,3.81 70.1,0.76 81.41,0.76 82.55,1.91 82.55,3.81 J8.12 82.04,6.86 78.49,6.86 76.58,8.76 75.06,8.76 71.37,12.45 JP8.2
RPD1/SCK1/RD1  (via drill 0.23 pad 0.43)
  Top 0.127: v59.18,38.23 59.18,36.2 58.9,35.91 IC1.76
  Bottom 0.127: J10.11 69.85,49.53 69.85,47.62 69.22,46.99 69.22,43.94 66.55,41.27 63.25,41.27 60.2,38.23 v59.18,38.23
RPD10/SCK4/RD10  (via drill 0.23 pad 0.43)
  Top 0.127: IC3.34 27.43,30.86 v28.19,30.1 | v56.77,26.54 56.77,29.72 57.78,30.73 59.05,30.73 59.18,30.61 59.82,30.61 59.93,30.72 IC1.69
  Bottom 0.127: v28.19,30.1 30.61,30.1 31.24,29.46 37.97,29.46 41.91,25.53 55.37,25.53 56.39,26.54 v56.77,26.54
SQICS0/RPD4/RD4  (via drill 0.23 pad 0.43)
  Top 0.127: v69.85,43.81 70.1,44.07 76.83,44.07 77.98,45.21 81.15,45.21 81.28,45.34 v81.41,45.34 | IC1.81 56.9,35.95 57.4,36.45 57.4,37.59 v57.53,37.72
  Bottom 0.127: v57.53,37.72 60.2,37.72 63.37,40.89 66.93,40.89 v69.85,43.81 | v81.41,45.34 v81.4,45.34 R24.1
SQICS1/RPD5/RD5  (via drill 0.23 pad 0.43)
  Top 0.127: IC1.82 56.5,35.93 57.02,36.45 57.02,38.86 v57.66,39.5
  Bottom 0.127: J7.2 61.85,48.26 59.69,46.1 59.69,43.18 58.04,41.53 58.04,40.01 57.66,39.62 v57.66,39.5
TCK/EBIA19/AN29/RA1  (via drill 0.23 pad 0.43)
  Top 0.127: IC1.38 54.1,20.83 54.86,20.07 54.86,19.43 53.72,18.29 v53.72,17.91
  Bottom 0.127: JP3.4 58.09,8.13 54.99,8.13 53.72,9.4 v53.72,17.91
TDI/EBIA18/AN30/RPF13/SCK5/RF13  (via drill 0.23 pad 0.43)
  Top 0.127: v54.36,17.91 54.36,18.41 55.24,19.3 55.24,20.07 54.5,20.81 IC1.39
  Bottom 0.127: v54.36,17.91 54.36,12.06 54.99,11.43 54.99,10.11 JP3.2
TDO/EBIA17/AN31/RPF12/RF12  (via drill 0.23 pad 0.43)
  Top 0.127: v54.99,17.91 54.99,18.54 55.5,19.05 55.5,20.19 54.9,20.79 IC1.40
  Bottom 0.127: v54.99,17.91 54.99,13.46 57.4,11.05 JP3.3
TMS/EBIA16/AN24/RA0
  Top 0.127: IC1.17 45.39,26.72 43.18,24.51 43.18,18.72 JP3.1
TRCLK/SQICLK/RA6  (via drill 0.23 pad 0.43)
  Top 0.127: IC1.89 53.7,34.14 53.59,34.04 52.07,34.04 51.94,33.91 v50.04,33.91
  Bottom 0.127: JP4.1 46.74,37.72 50.04,34.42 v50.04,33.91
TRD0/SQID0/RG13
  Top 0.127: IC1.97 50.5,35.86 50.16,36.2 50.16,36.7 49.28,37.59 JP4.2
TRD1/SQID1/RG12
  Top 0.127: IC1.96 50.9,35.84 50.55,36.2 50.55,36.83 50.42,36.96 50.42,39.55 JP4.3
TRD2/SQID2/RG14
  Top 0.127: IC1.95 51.3,35.82 50.8,36.32 50.8,38.48 52.2,39.88 53.47,39.88 54.36,40.77 JP4.4
TRD3/SQID3/RA7
  Top 0.127: IC1.90 53.3,36.03 53.47,36.2 53.47,37.72 56.39,40.64 56.64,40.64 56.9,40.89 JP4.5
USB5V0  (via drill 0.23 pad 0.43)
  Bottom 0.127: R1.2 v10.03,27.56
  Bottom 0.254: IC2.19 13.22,26.92 C9.1 12.96,27.68 v12.95,27.69 | v12.7,29.34 12.7,28.97 C7.1 13.34,29.07 v13.34,29.34
  other vias: 6.99,26.8 6.48,27.3 8.51,27.3 7.49,27.3 8,26.8
  pour Top (no thermals): 6.22,25.91 9.02,25.91 9.02,27.43 6.22,27.43
  pour Route15 (isolate 0.305, rank 2, no thermals): 5.46,30.35 13.34,30.35 14.22,29.46 14.22,24.51 27.05,11.68 35.31,11.68 37.47,9.53 37.47,6.86 36.96,6.35 26.67,6.35 18.16,14.86 5.46,14.86
USB_D+  (via drill 0.23 pad 0.43)
  Top 0.203: v83.06,17.65 82.93,17.53 76.69,17.53 J12.3 75.71,17.53 75.06,17.53 72.77,19.81 66.67,19.81 64.52,21.97 64.52,24.38 63.63,25.27 62.1,25.27 61.95,25.12 IC1.55
  Bottom 0.203: J11.3 83.69,17.02 v83.06,17.65
USB_D-  (via drill 0.23 pad 0.43)
  Top 0.203: v83.82,17.65 83.19,17.02 77.2,17.02 J12.2 75.07,17.14 74.8,17.14 72.52,19.43 66.42,19.43 64.14,21.72 64.14,24.13 63.37,24.89 62.23,24.89 62.06,24.72 IC1.54
  Bottom 0.203: J11.2 83.83,17.67
  Bottom 0.254: 83.83,17.67 v83.82,17.65
USBID/RPF3/RF3  (via drill 0.23 pad 0.43)
  Top 0.127: IC1.56 59.94,25.52 59.56,25.15 59.56,23.5 59.94,23.11 60.45,23.11 66.8,16.76 66.8,16.13 68.58,14.35 74.68,14.35 75.06,14.73 78.36,14.73 78.87,15.24 82.17,15.24 v83.44,16.51
  Bottom 0.127: J11.4 84.66,16.38 83.69,16.38 83.57,16.51 v83.44,16.51
VBUS  (via drill 0.23 pad 0.43)
  Top 0.203: IC1.51 61.31,23.52 v61.72,23.11
  Bottom 0.203: 62.61,22.99 61.85,22.99 | 62.87,22.73 64.64,20.95 68.58,20.95 JP6.2
  Bottom 0.254: 61.85,22.99 v61.72,23.11 | 62.61,22.99 62.87,22.73
  Bottom 0.61: IC4.1 82.74,19.49 arc-90 v83.44,18.8
  other vias: 40.89,3.56 41.91,3.56 42.93,3.56 41.4,2.92 42.42,2.92 83.82,19.43 84.71,19.43 84.33,18.8 85.22,18.8
  pour Bottom (no thermals): 85.47,18.16 85.47,19.68 83.06,19.68 83.06,18.16
  pour Top (no thermals): 37.85,7.87 38.35,8.38 39.75,8.38 40.13,8 40.13,6.73 43.18,3.68 43.18,2.54 41.27,2.54 37.85,5.97
  pour Route15 (isolate 0.305, rank 2, no thermals): 39.37,3.94 39.37,2.67 41.66,0.38 87.76,0.38 88.52,1.14 88.52,27.3 72.01,27.18 68.58,24 68.58,21.08 71.12,21.08 71.25,23.11 72.26,24 74.17,24 74.8,23.37 75.56,22.48 77.47,20.7 82.68,20.7 83.31,19.81 83.31,8.38 79.25,4.32 69.85,4.32 67.06,1.52 45.59,1.52 43.18,3.94
VCC3V3  (via drill 0.23 pad 0.43)
  Top 0.127: LD2.A v80.52,39.24 | LD1.A v78.74,39.24 | LD3.A v82.3,39.24 | LD4.A v84.07,39.24 | R22.2 v22.48,18.92
  Top 0.203: IC7.1 IC7.4
  Top 0.254: IC3.29 C21.1 v21.09,29.98 v21.08,29.97 | IC3.17 v9.65,51.56 | v54.1,19.43 v54.09,19.44 C6.1 53.7,20.33 IC1.37 | v21.21,3.68 21.67,4.14 J13.4 | v51.69,37.08 51.69,36.82 C3.1 52.1,36.17 IC1.93 | IC1.83 56.1,36.3 C2.1 56.39,36.82 v56.39,37.08 | v62.99,23.37 62.6,23.37 C1.1 61.81,23.92 IC1.52 | v62.99,27.69 62.6,27.69 C10.1 62.13,27.92 IC1.62 | C4.1 45.72,27.56 | 45.72,27.56 46.1,27.94 47.38,27.94 IC1.14 | 45.72,27.56 45.59,27.69 v45.21,27.69 | IC1.46 57.3,20.67 C8.1 57.78,19.69 v57.78,19.43 | IC1.74 61.77,32.72 v61.85,32.64
  Top 0.305: v57.78,18.67 C17.1 58.16,18.03 58.61,18.48 IC7.4
  Top 1.016: J5.2 50.8,3.05 51.94,4.19 55.37,4.19 55.63,4.45
  Bottom 0.127: R14.2 v21.09,51.3 v21.08,51.31 | R20.2 v12.45,32.52 v12.45,32.51 | R21.2 27.42,33.39 27.43,33.4 v27.43,33.53 | R16.2 v80.26,16.26 | R19.2 v10.67,32.51 | R18.2 17.78,32.77 v17.78,32.51 | R5.2 37.72,41.78 v37.59,41.91
  Bottom 0.254: R40.2 34.29,22.35 34.04,22.61 31.88,22.61 v31.5,22.23 | C23.1 v9.64,51.55 v9.65,51.56 | v17.91,49.78 17.54,49.78 C25.1 17.91,48.91 v17.91,48.9 | v3.81,34.67 3.44,34.67 C26.1 3.06,34.27 3.43,33.91 v3.81,33.91 | C27.1 21.07,3.55 v21.21,3.68 | D1.2 50.78,26.91 v50.8,26.92 | C12.1 61.33,32.64 v61.85,32.64
  other vias: 29.72,22.23 30.61,22.23 31.5,21.34 31.5,20.45 31.5,19.56 48.64,21.34 48.13,21.84 47.62,21.34
  pour Bottom (isolate 0.305, rank 3, no thermals): 23.5,22.48 23.5,19.3 31.75,19.3 31.75,22.48
  pour Top (no thermals): 47.37,22.1 47.37,20.19 48.9,20.19 48.9,22.1
  pour Route15 (isolate 0.305, rank 3): 0,11.18 12.57,11.18 12.57,0 21.46,0 21.46,6.48 27.05,12.06 48.26,12.06 50.04,10.41 50.04,5.59 50.42,5.21 64.01,5.21 67.56,8.76 79.38,8.76 80.52,9.91 80.52,17.65 79.5,18.67 72.9,18.67 70.87,20.7 65.91,20.7 65.66,20.95 65.66,23.5 69.85,27.69 88.52,27.69 88.52,52.96 8.26,52.96 8.26,50.93 11.81,50.93 11.81,35.94 0,35.94
  pour Top (no thermals): 54.74,2.16 55.12,1.78 56.64,1.78 56.9,2.03 56.9,6.48 56.77,6.6 54.86,6.6 54.74,6.48
VCC5V0  (via drill 0.23 pad 0.43)
  other vias: 78.11,19.94 79.5,19.94 78.11,19.18 79.5,19.18
  pour Route15 (isolate 0.305, no thermals): 44.32,10.41 44.83,10.92 46.86,10.92 49.53,8.26 49.53,5.21 49.91,4.83 59.69,4.83 59.69,6.86 61.98,6.86 61.98,4.7 63.88,4.7 67.69,8.38 79.63,8.38 80.9,9.65 80.9,17.91 79.88,18.92 77.47,18.92 77.47,20.32 82.55,20.32 82.93,19.81 82.93,8.51 79.12,4.7 69.72,4.7 66.93,1.91 46.74,1.91 44.07,4.45 44.07,8.13 44.32,8.38
  pour Bottom (rank 2, no thermals): 77.47,20.19 77.47,18.92 79.76,18.92 79.76,20.19
VCCSHIELD
  Top 0.813: JP9.2 J5.5
VEXT
  Top 0.889: J16.1 35.18,5.97 36.58,5.97 41.53,1.02 64.52,1.02 J5.8
  Top 1.524: J15.1 10.52,10.69 9.02,12.19 4.32,12.19 3.05,13.46 J14.1
  Bottom 1.27: J16.1 33.66,7.37 33.27,6.99 30.1,6.99 21.08,16 16.38,16 16,15.62 12.83,15.62 10.52,13.31 J15.1
  pour Top (no thermals): 9.53,9.65 9.53,5.59 10.03,5.08 10.92,5.08 11.43,5.59 11.43,9.65 10.92,10.16 10.03,10.16
  pour Bottom (no thermals): 10.03,5.08 9.53,5.59 9.53,9.65 10.03,10.16 10.92,10.16 11.43,9.65 11.43,5.59 10.92,5.08
  pour Route2 (no thermals): 9.53,9.65 10.03,10.16 10.92,10.16 11.43,9.65 11.43,5.59 10.92,5.08 10.03,5.08 9.53,5.59
  pour Route15 (no thermals): 9.53,9.65 9.53,5.59 10.03,5.08 10.92,5.08 11.43,5.59 11.43,9.65 10.92,10.16 10.03,10.16
VREF+/CVREF+/AN28/AERXD3/RA10  (via drill 0.23 pad 0.43)
  Top 0.127: v52.45,27.56 52.45,26.29 50.5,24.34 IC1.29
  Bottom 0.127: J7.15 44.07,50.8 42.67,49.4 42.67,47.5 40.77,45.59 40.77,38.48 43.31,35.94 43.31,34.04 47.5,29.84 48.39,29.84 49.4,28.83 50.8,28.83 52.07,27.56 v52.45,27.56
VREF-/CVREF-/AN27/AERXD2/RA9  (via drill 0.23 pad 0.43)
  Top 0.127: IC1.28 50.1,24.45 51.94,26.29 v51.94,28.45
  Bottom 0.127: J7.16 44.2,46.74 43.69,46.23 43.69,40.01 43.81,39.88 43.81,34.29 47.88,30.23 48.51,30.23 49.66,29.08 51.31,29.08 v51.94,28.45
VRIN
  pour Bottom (isolate 0.305, rank 3, no thermals): 19.43,4.06 19.43,6.48 22.1,6.48 22.1,5.59 22.61,5.08 32.38,5.08 33.66,6.35 40.39,6.35 42.16,8.13 43.81,8.13 43.81,5.97 42.16,4.32 41.91,4.32 34.54,4.32 34.29,4.06
VROUT  (via drill 0.23 pad 0.43)
  other vias: 17.4,11.81 18.29,11.81 19.18,11.81 17.4,11.05 18.29,11.05 19.18,11.05
  pour Bottom (isolate 0.305, no thermals): 15.49,14.99 21.08,14.99 21.08,11.3 24,11.3 24,10.54 22.61,10.54 22.61,9.65 20.45,9.65 20.19,9.4 20.19,6.86 18.16,6.86 18.16,8.89 17.65,9.4 15.49,9.4
  pour Route15 (isolate 0.305, no thermals): 17.02,12.19 17.02,8.89 21.72,4.19 41.53,4.19 42.29,4.95 42.29,8.13 42.93,8.76 43.43,8.76 43.81,9.14 43.81,10.41 43.31,10.92 41.78,10.92 40.51,9.65 40.51,7.24 39.24,5.97 26.42,5.97 17.78,14.61 17.02,14.61
VU
  Bottom 0.254: J16.2 33.27,9.91 32.64,9.27 32.38,9.27 R35.2
  pour Bottom (no thermals): 32.77,10.29 32.77,9.4 33.4,8.76 39.24,8.76 39.62,8.38 43.94,8.38 44.45,7.87 44.45,6.73 44.83,6.35 46.1,6.35 46.48,6.73 46.48,9.02 43.94,11.56 34.04,11.56
  pour Bottom (isolate 0.305, no thermals): 37.08,16.89 37.08,14.99 34.92,14.99 34.8,14.86 34.8,11.81 35.05,11.56 35.05,10.92 33.4,10.92 33.4,14.99 33.02,14.99 33.02,16.89

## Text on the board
tPlace: 1 | SCL | SDA | A | G | 9 | 8 | 7 | 6 | 5 | 4 | 3 | 2 | 1 | 0 | 13 | 12 | 11 | 10 | TX | RX | 31 | 30 | 41 | 40 | 39 | 38 | 37 | 36 | 35 | 34 | 33 | 32 | 29 | 28 | 27 | 26 | 1 | GND | RESET | SPI | 1 | SPI | SELECT | ICSP | (AIN12) | 1 | USB | UART | AB | A | 1 | GND | + | - | 15V MAX! | EXT | UART | USB | LDO | OUT | 5V0 | GND | 1 | JTAG | A6 | A7 | A8 | A10 | A11 | 3V3 | 5V0 | A0 | A1 | A2 | A3 | A9 | A4 | A5 | 1 | 1 | VU SELECT | EN | ANALOG | IN | VU | IOREF | RST | GND | VIN | LDO | NC | + | _
bPlace: PB200-302 | REV B | 3V3 | 5V0 | GND | 3V3 | NC | 5V0
Measures: Slot Drills | 0.026 x 0.125"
